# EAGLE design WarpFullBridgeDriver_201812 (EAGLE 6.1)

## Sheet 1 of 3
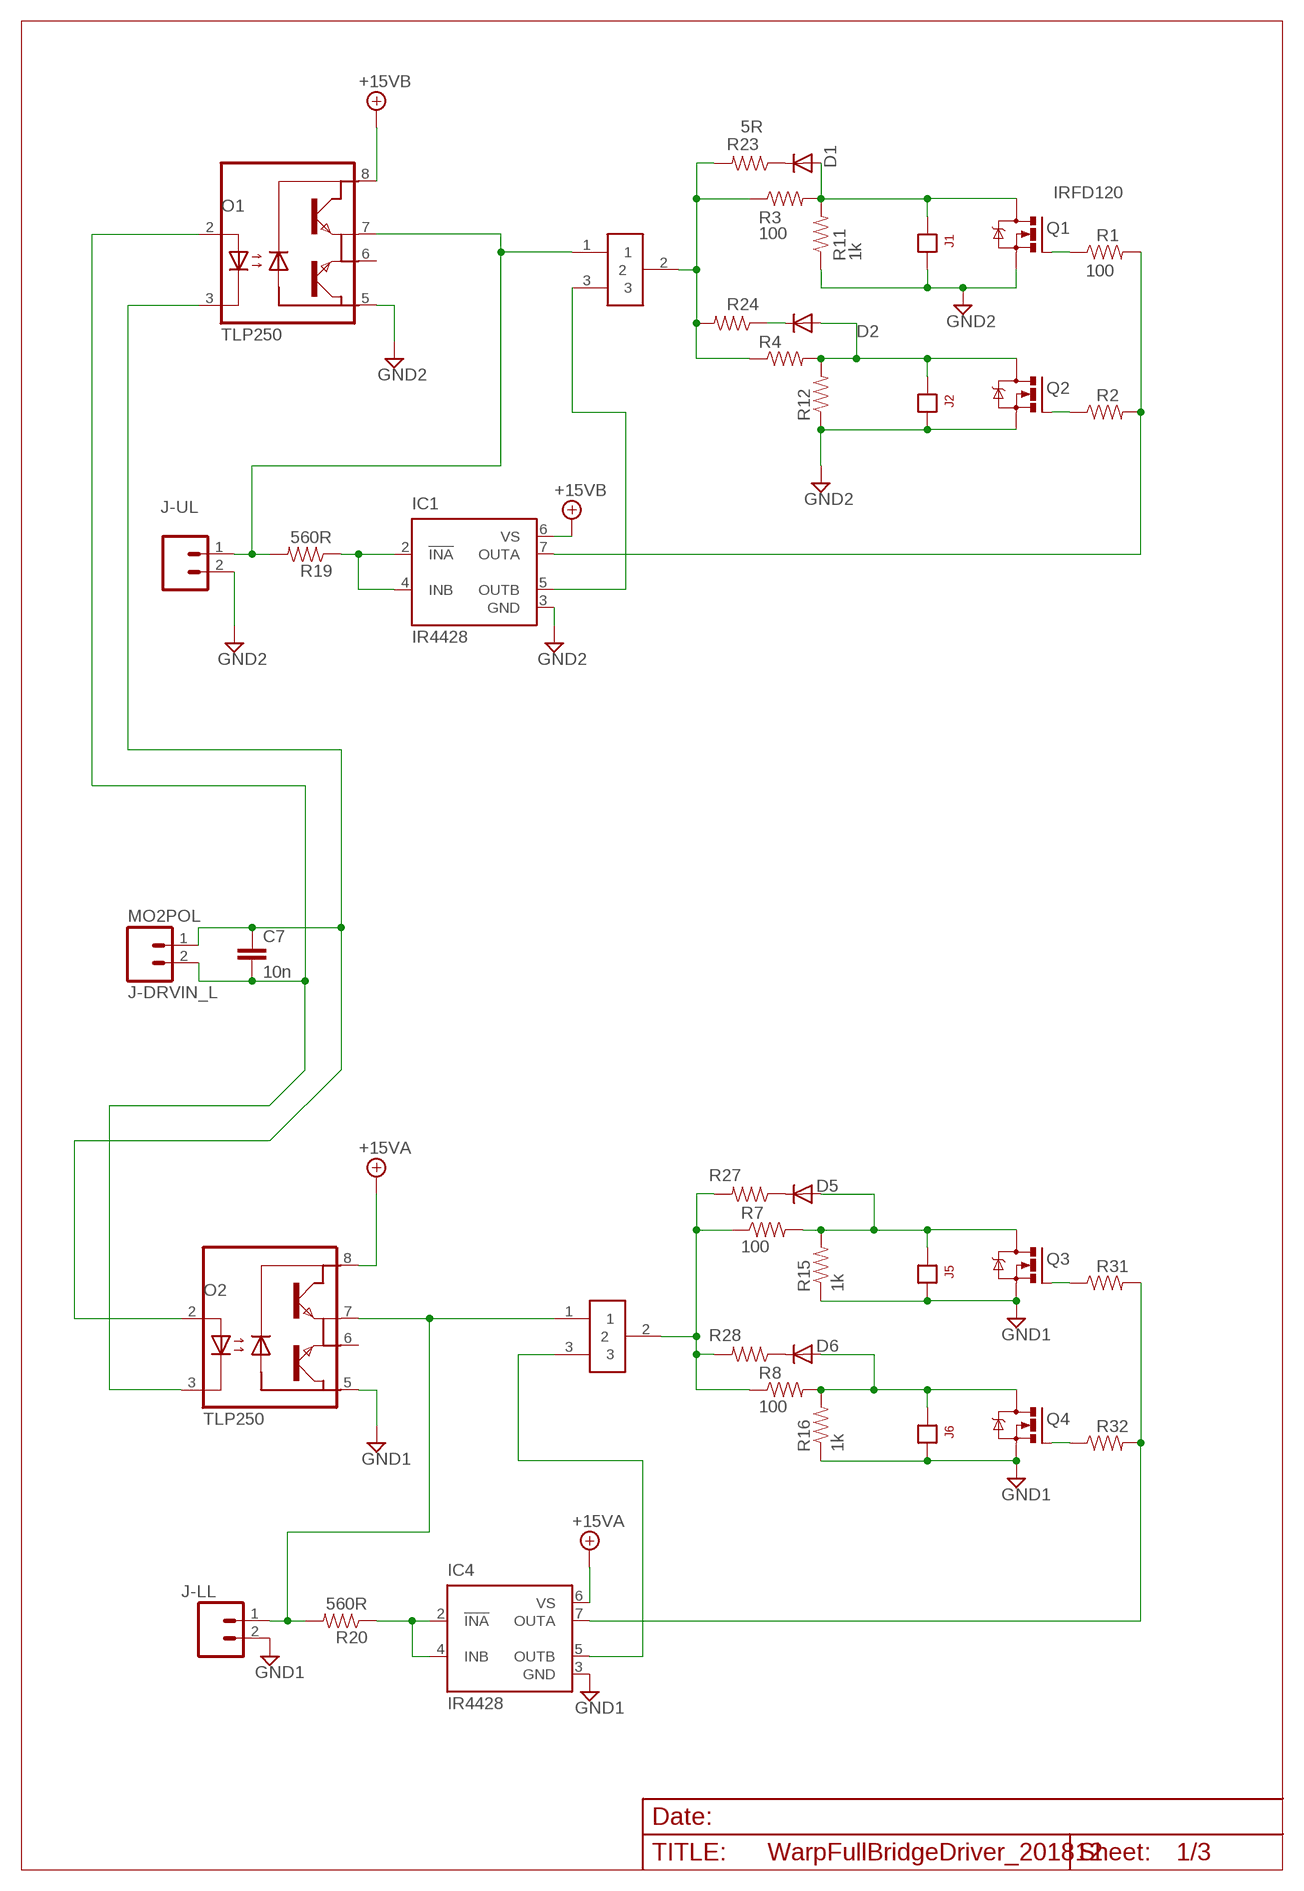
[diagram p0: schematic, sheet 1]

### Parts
C7  10n  BCAP  [BCAP]
D1  1N4148DO35-7  [D3]
D2  1N4148DO35-7  [D3]
D5  1N4148DO35-7  [D3]
D6  1N4148DO35-7  [D3]
IC1  IR4428  [DIL08]
IC4  IR4428  [DIL08]
J1  JP1  [JP1]
J2  JP1  [JP1]
J5  JP1  [JP1]
J6  JP1  [JP1]
J-DRVIN_L  MO2POL  [MOLEX-1X2]
J-LL  MO2POL  [MOLEX-1X2]
J-UL  MO2POL  [MOLEX-1X2]
JP1  JP1X3  [JP1X3]
JP2  JP1X3  [JP1X3]
O1  TLP250  TLP250DIP8-L39  [DIL08-L39]
O2  TLP250  TLP250DIP8-L39  [DIL08-L39]
Q1  IRFD120  [DIL04]
Q2  IRFD120  [DIL04]
Q3  IRFD120  [DIL04]
Q4  IRFD120  [DIL04]
R1  100  RESISTORPTH-1/4W  [AXIAL-0.4]
R2  100  RESISTORPTH-1/4W  [AXIAL-0.4]
R3  100  RESISTORPTH-1/4W  [AXIAL-0.4]
R4  100  RESISTORPTH-1/4W  [AXIAL-0.4]
R7  100  RESISTORPTH-1/4W  [AXIAL-0.4]
R8  100  RESISTORPTH-1/4W  [AXIAL-0.4]
R11  1k  R4  [AXIAL-0.4]
R12  1k  R4  [AXIAL-0.4]
R15  1k  R4  [AXIAL-0.4]
R16  1k  R4  [AXIAL-0.4]
R19  560R  R4  [AXIAL-0.4]
R20  560R  R4  [AXIAL-0.4]
R23  5R  R4  [AXIAL-0.4]
R24  5R  R4  [AXIAL-0.4]
R27  5R  R4  [AXIAL-0.4]
R28  5R  R4  [AXIAL-0.4]
R31  100  RESISTORPTH-1/4W  [AXIAL-0.4]
R32  100  RESISTORPTH-1/4W  [AXIAL-0.4]

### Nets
+15VA: IC4.6(VS) O2.8(VCC) ; also sheet 3
+15VB: IC1.6(VS) O1.8(VCC) ; also sheet 3
GND1: IC4.3(GND) J5.2 J6.2 J-LL.2 O2.5(GND) Q3.4(S) Q4.4(S) R15.P$1 R16.P$1 ; also sheet 3
GND2: IC1.3(GND) J1.2 J2.2 J-UL.2 O1.5(GND) Q1.4(S) Q2.4(S) R11.P$1 R12.P$1 ; also sheet 3
N$1: J-LL.1 JP2.1 O2.7(VO2) R20.P$2
N$2: D2.A J2.1 Q2.1(D) R4.P$2 R12.P$2
N$3: D1.A J1.1 Q1.1(D) R3.P$2 R11.P$2
N$4: D1.C R23.P$1
N$5: J-UL.1 JP1.1 O1.7(VO2) R19.P$2
N$6: IC1.2(!INA) IC1.4(INB) R19.P$1
N$7: Q1.3(G) R1.P$1
N$8: D6.A J6.1 Q4.1(D) R8.P$2 R16.P$2
N$11: C7.1 J-DRVIN_L.1 O1.3(C) O2.2(A)
N$12: D5.A J5.1 Q3.1(D) R7.P$2 R15.P$2
N$15: IC1.7(OUTA) R1.P$2 R2.P$2
N$16: C7.2 J-DRVIN_L.2 O1.2(A) O2.3(C)
N$17: Q2.3(G) R2.P$1
N$21: D2.C R24.P$1
N$23: JP2.2 R7.P$1 R8.P$1 R27.P$2 R28.P$2
N$27: IC1.5(OUTB) JP1.3
N$28: D5.C R27.P$1
N$29: IC4.7(OUTA) R31.P$2 R32.P$2
N$30: IC4.2(!INA) IC4.4(INB) R20.P$1
N$31: D6.C R28.P$1
N$32: IC4.5(OUTB) JP2.3
N$36: JP1.2 R3.P$1 R4.P$1 R23.P$2 R24.P$2
N$39: Q3.3(G) R31.P$1
N$41: Q4.3(G) R32.P$1
Unconnected: O1.6(VO) O2.6(VO)

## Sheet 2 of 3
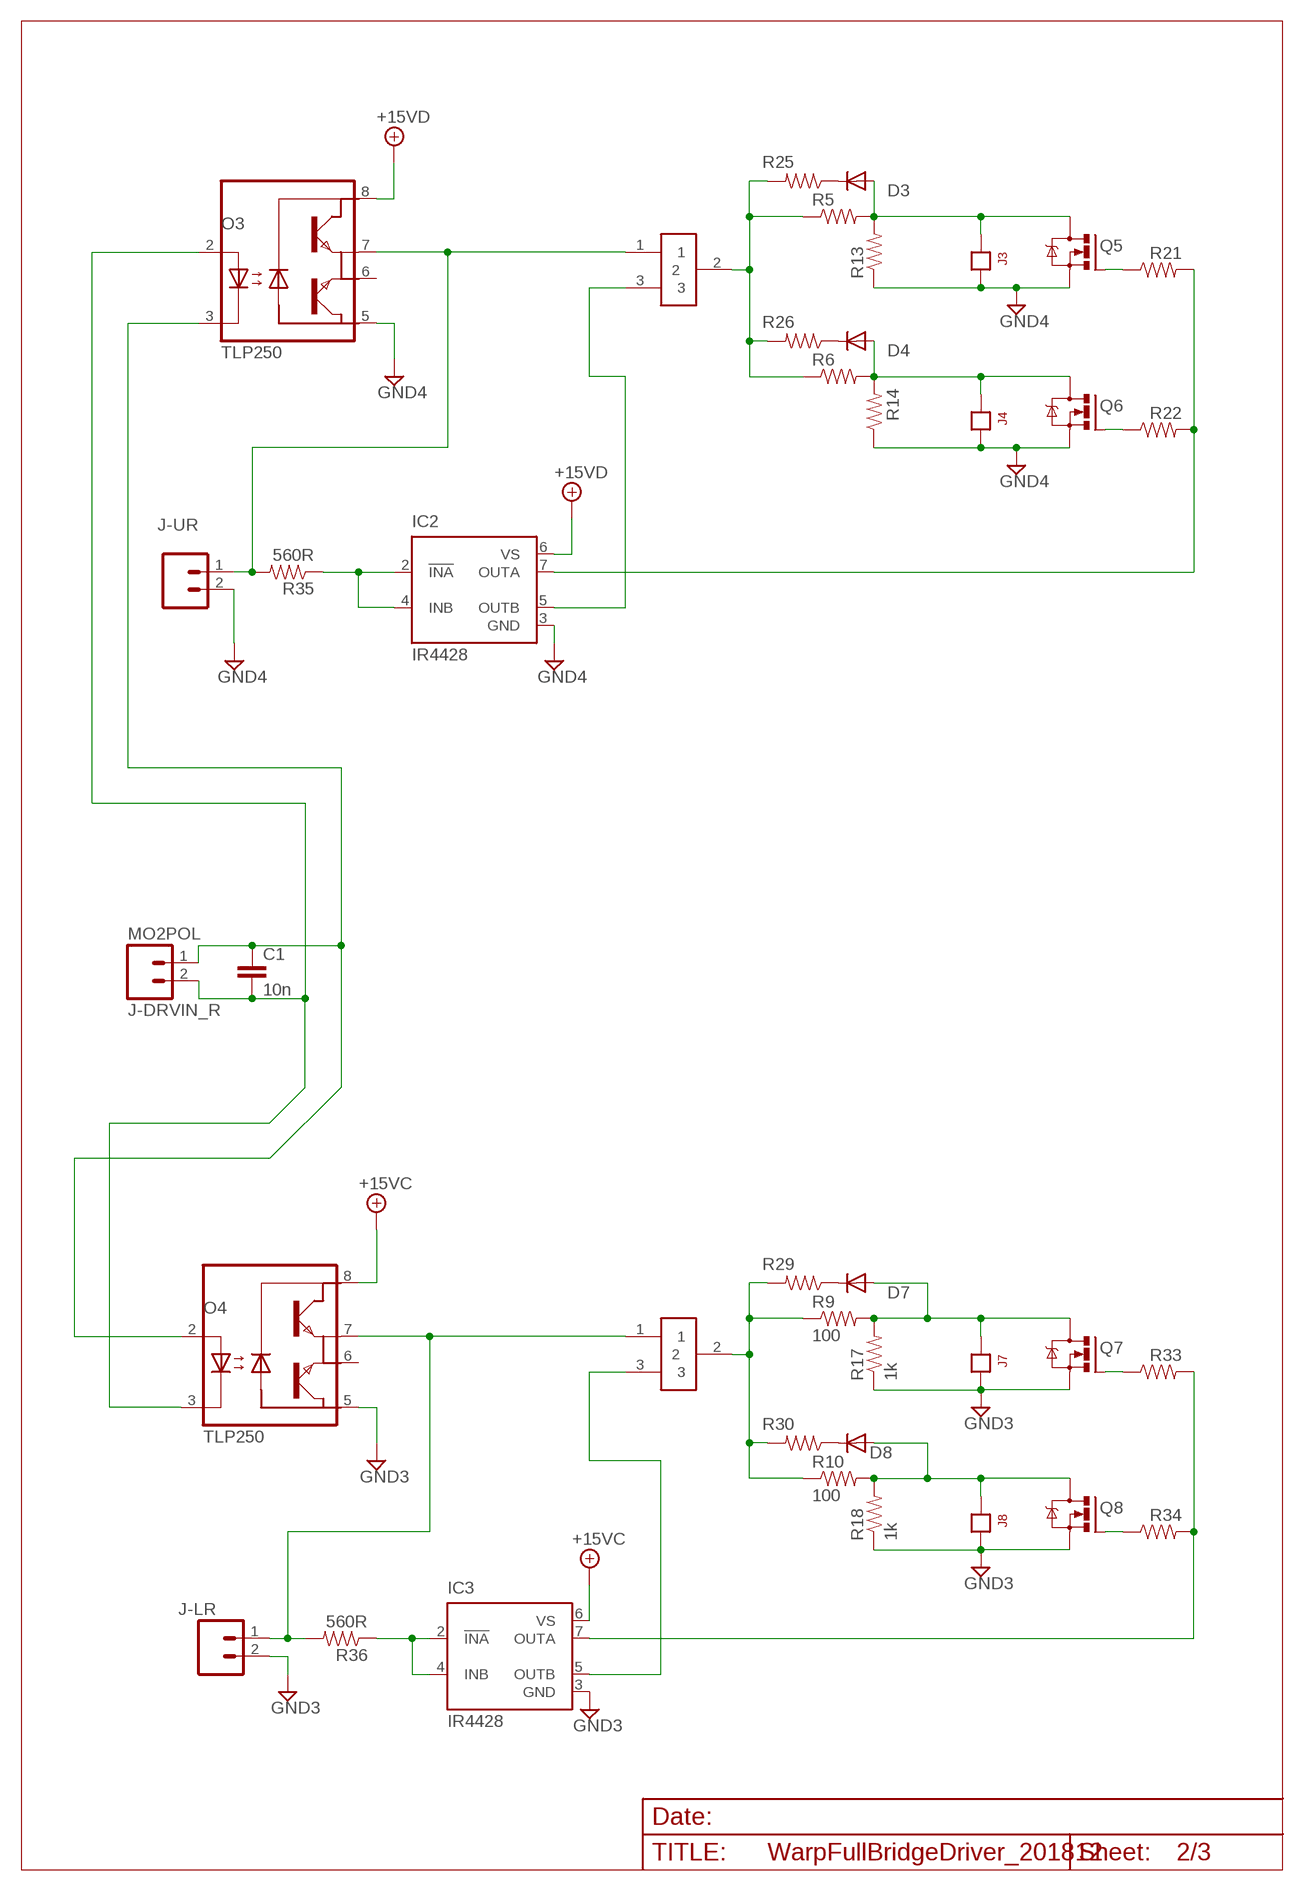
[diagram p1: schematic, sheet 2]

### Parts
C1  10n  BCAP  [BCAP]
D3  1N4148DO35-7  [D3]
D4  1N4148DO35-7  [D3]
D7  1N4148DO35-7  [D3]
D8  1N4148DO35-7  [D3]
IC2  IR4428  [DIL08]
IC3  IR4428  [DIL08]
J3  JP1  [JP1]
J4  JP1  [JP1]
J7  JP1  [JP1]
J8  JP1  [JP1]
J-DRVIN_R  MO2POL  [MOLEX-1X2]
J-LR  MO2POL  [MOLEX-1X2]
J-UR  MO2POL  [MOLEX-1X2]
JP3  JP1X3  [JP1X3]
JP4  JP1X3  [JP1X3]
O3  TLP250  TLP250DIP8-L39  [DIL08-L39]
O4  TLP250  TLP250DIP8-L39  [DIL08-L39]
Q5  IRFD120  [DIL04]
Q6  IRFD120  [DIL04]
Q7  IRFD120  [DIL04]
Q8  IRFD120  [DIL04]
R5  100  RESISTORPTH-1/4W  [AXIAL-0.4]
R6  100  RESISTORPTH-1/4W  [AXIAL-0.4]
R9  100  RESISTORPTH-1/4W  [AXIAL-0.4]
R10  100  RESISTORPTH-1/4W  [AXIAL-0.4]
R13  1k  R4  [AXIAL-0.4]
R14  1k  R4  [AXIAL-0.4]
R17  1k  R4  [AXIAL-0.4]
R18  1k  R4  [AXIAL-0.4]
R21  100  RESISTORPTH-1/4W  [AXIAL-0.4]
R22  100  RESISTORPTH-1/4W  [AXIAL-0.4]
R25  5R  R4  [AXIAL-0.4]
R26  5R  R4  [AXIAL-0.4]
R29  5R  R4  [AXIAL-0.4]
R30  5R  R4  [AXIAL-0.4]
R33  100  RESISTORPTH-1/4W  [AXIAL-0.4]
R34  100  RESISTORPTH-1/4W  [AXIAL-0.4]
R35  560R  R4  [AXIAL-0.4]
R36  560R  R4  [AXIAL-0.4]

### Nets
+15VC: IC3.6(VS) O4.8(VCC) ; also sheet 3
+15VD: IC2.6(VS) O3.8(VCC) ; also sheet 3
GND3: IC3.3(GND) J7.2 J8.2 J-LR.2 O4.5(GND) Q7.4(S) Q8.4(S) R17.P$1 R18.P$1 ; also sheet 3
GND4: IC2.3(GND) J3.2 J4.2 J-UR.2 O3.5(GND) Q5.4(S) Q6.4(S) R13.P$1 R14.P$1 ; also sheet 3
N$9: D3.A J3.1 Q5.1(D) R5.P$2 R13.P$2
N$10: D4.A J4.1 Q6.1(D) R6.P$2 R14.P$2
N$13: D7.A J7.1 Q7.1(D) R9.P$2 R17.P$2
N$14: D8.A J8.1 Q8.1(D) R10.P$2 R18.P$2
N$18: IC2.7(OUTA) R21.P$2 R22.P$2
N$19: Q5.3(G) R21.P$1
N$22: Q6.3(G) R22.P$1
N$24: D3.C R25.P$1
N$25: D4.C R26.P$1
N$26: J-UR.1 JP3.1 O3.7(VO2) R35.P$2
N$33: IC2.5(OUTB) JP3.3
N$34: D7.C R29.P$1
N$35: J-LR.1 JP4.1 O4.7(VO2) R36.P$2
N$37: D8.C R30.P$1
N$38: IC3.5(OUTB) JP4.3
N$40: JP3.2 R5.P$1 R6.P$1 R25.P$2 R26.P$2
N$43: Q7.3(G) R33.P$1
N$44: IC2.2(!INA) IC2.4(INB) R35.P$1
N$45: Q8.3(G) R34.P$1
N$46: IC3.7(OUTA) R33.P$2 R34.P$2
N$47: C1.1 J-DRVIN_R.1 O3.3(C) O4.2(A)
N$48: C1.2 J-DRVIN_R.2 O3.2(A) O4.3(C)
N$49: JP4.2 R9.P$1 R10.P$1 R29.P$2 R30.P$2
N$51: IC3.2(!INA) IC3.4(INB) R36.P$1
Unconnected: O3.6(VO) O4.6(VO)

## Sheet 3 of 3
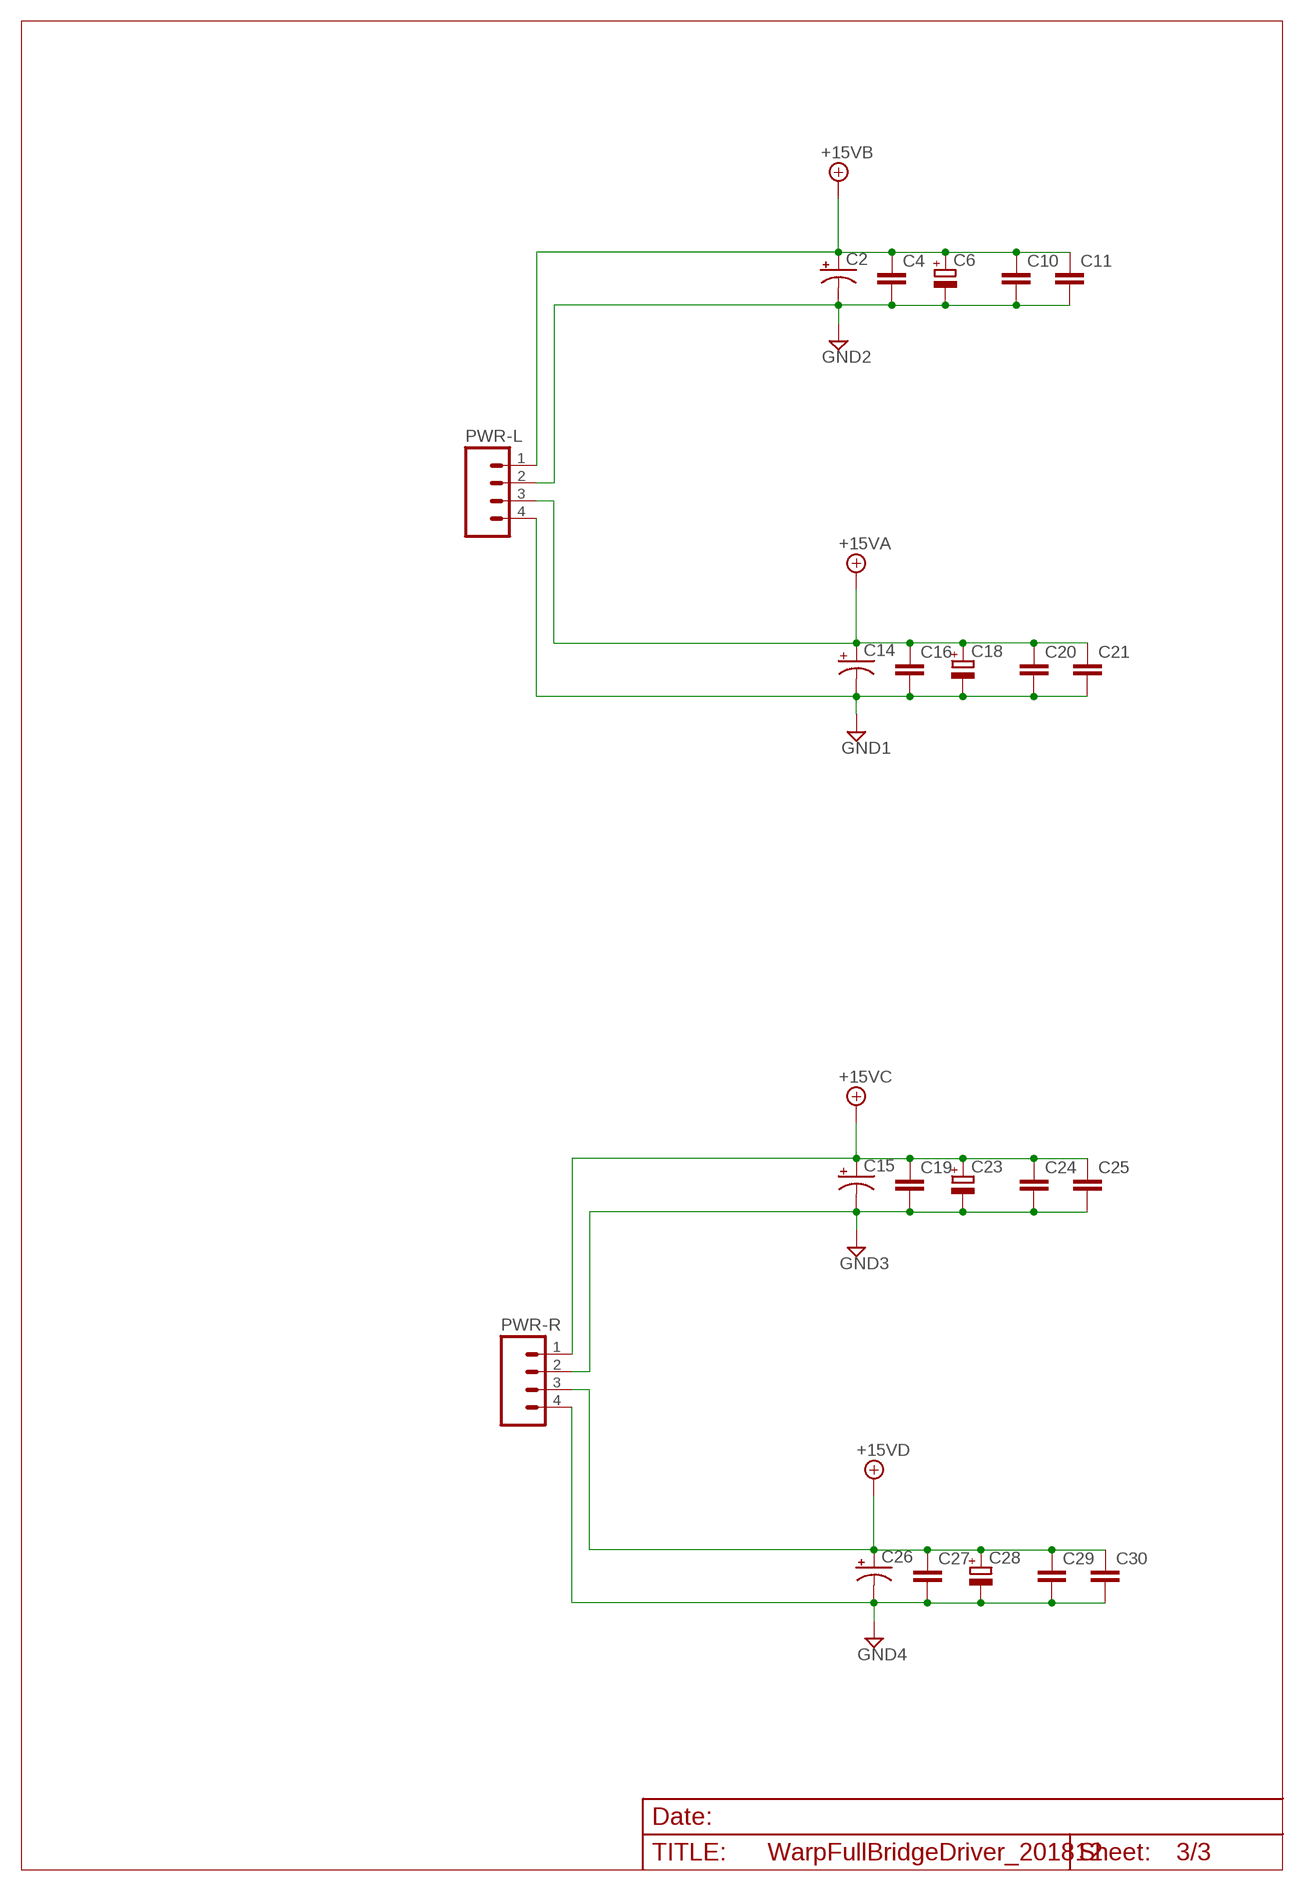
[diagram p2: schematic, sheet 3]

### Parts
C2  CAP_POLPTH1  [CPOL-RADIAL-100UF-25V]
C4  BCAP  [BCAP]
C6  C-RB200100  [CPOL-RADIAL-10UF-25V]
C10  BCAP  [BCAP]
C11  BCAP  [BCAP]
C14  CAP_POLPTH1  [CPOL-RADIAL-100UF-25V]
C15  CAP_POLPTH1  [CPOL-RADIAL-100UF-25V]
C16  BCAP  [BCAP]
C18  C-RB200100  [CPOL-RADIAL-10UF-25V]
C19  BCAP  [BCAP]
C20  BCAP  [BCAP]
C21  BCAP  [BCAP]
C23  C-RB200100  [CPOL-RADIAL-10UF-25V]
C24  BCAP  [BCAP]
C25  BCAP  [BCAP]
C26  CAP_POLPTH1  [CPOL-RADIAL-100UF-25V]
C27  BCAP  [BCAP]
C28  C-RB200100  [CPOL-RADIAL-10UF-25V]
C29  BCAP  [BCAP]
C30  BCAP  [BCAP]
PWR-L  MO4POL  [MOLEX-4]
PWR-R  MO4POL  [MOLEX-4]

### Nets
+15VA: C14.1(+) C16.1 C18.1(+) C20.1 C21.1 PWR-L.3 ; also sheet 1
+15VB: C2.1(+) C4.1 C6.1(+) C10.1 C11.1 PWR-L.1 ; also sheet 1
+15VC: C15.1(+) C19.1 C23.1(+) C24.1 C25.1 PWR-R.1 ; also sheet 2
+15VD: C26.1(+) C27.1 C28.1(+) C29.1 C30.1 PWR-R.3 ; also sheet 2
GND1: C14.2(-) C16.2 C18.2(-) C20.2 C21.2 PWR-L.4 ; also sheet 1
GND2: C2.2(-) C4.2 C6.2(-) C10.2 C11.2 PWR-L.2 ; also sheet 1
GND3: C15.2(-) C19.2 C23.2(-) C24.2 C25.2 PWR-R.2 ; also sheet 2
GND4: C26.2(-) C27.2 C28.2(-) C29.2 C30.2 PWR-R.4 ; also sheet 2

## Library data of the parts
C1 C7 = Andrew junk:BCAP
C2 C14 C15 C26 = SparkFun-Passives:CAP_POL: Capacitor Polarized
C4 C10 C11 C16 C19-C21 C24 C25 C27 C29 C30 = Andrew Misc:BCAP
C6 C18 C23 C28 = Andrew:C-RB200100
D1-D8 = Andrew Misc:1N4148: DIODE
IC1-IC4 = ir:IR4428: DUAL LOW SIDE DRIVER Source: ID4426.pdf; MF: INTERNATIONAL RECTIFIER(IR); MPN: IR4428PBF; OC_FARNELL: 1023268; OC_NEWARK: 19K8464
J1-J8 = Andrew Connectors:JP1
J-DRVIN_L J-DRVIN_R J-LL J-LR J-UL J-UR = Andrew_Connectors:MO2POL
JP1-JP4 = Andrew_Connectors:JP1X3
O1-O4 = Andrew IC:TLP250: HEWLETT PACKARD OPTO COUPLER
PWR-L PWR-R = Andrew_Connectors:MO4POL
Q1-Q8 = Andrew Transistor:IRFD120
R1-R10 R21 R22 R31-R34 = SparkFun-Passives:RESISTOR: Resistor
R11-R20 R23-R30 R35 R36 = Andrew Misc:R4

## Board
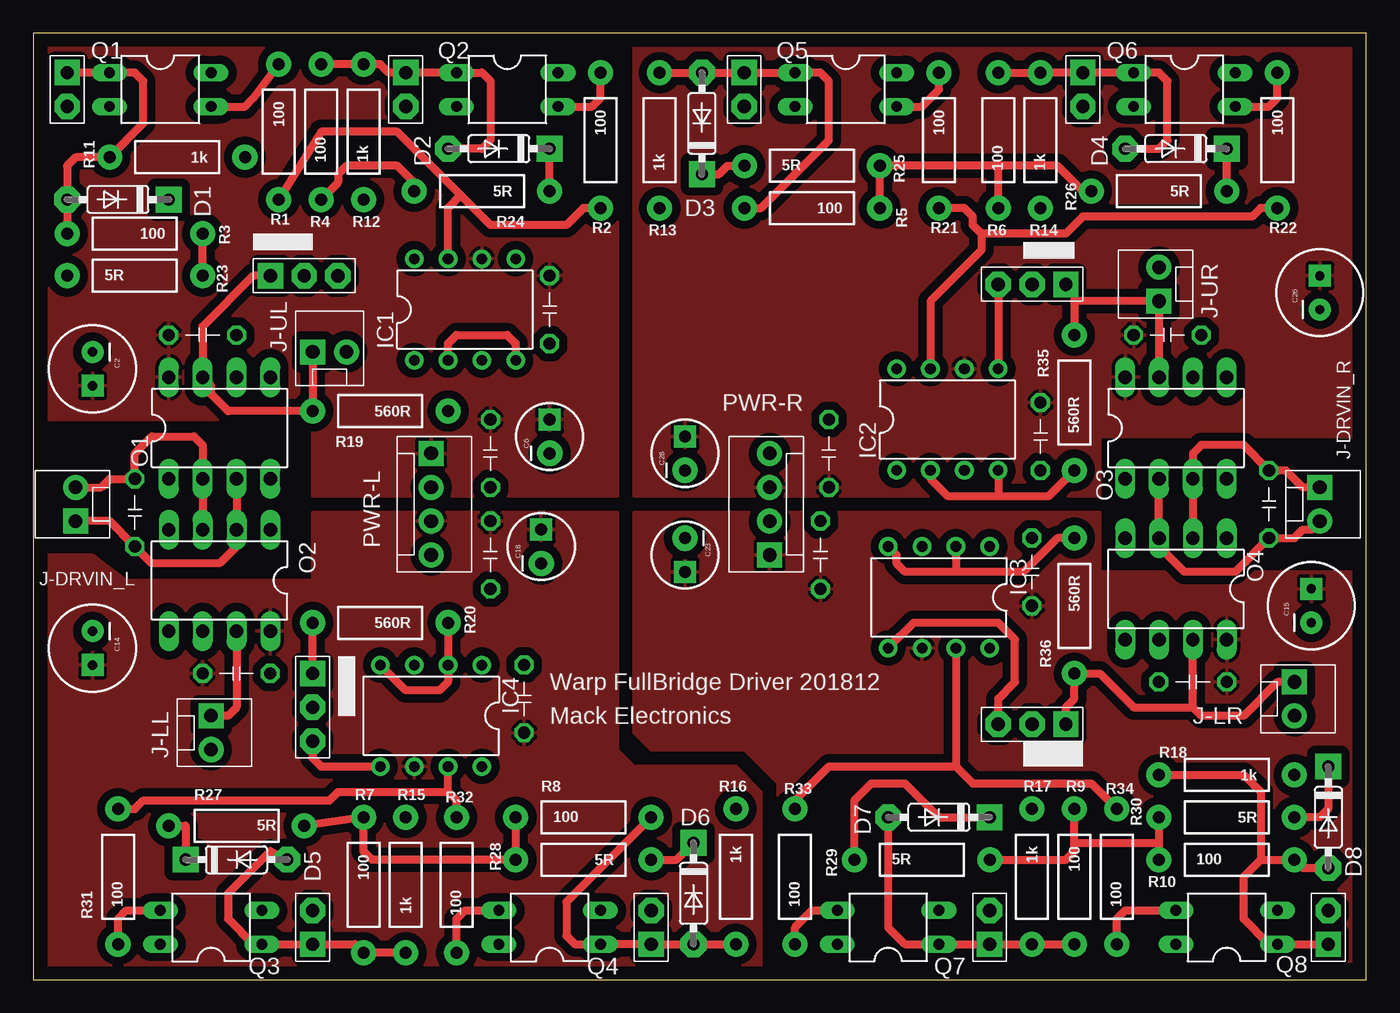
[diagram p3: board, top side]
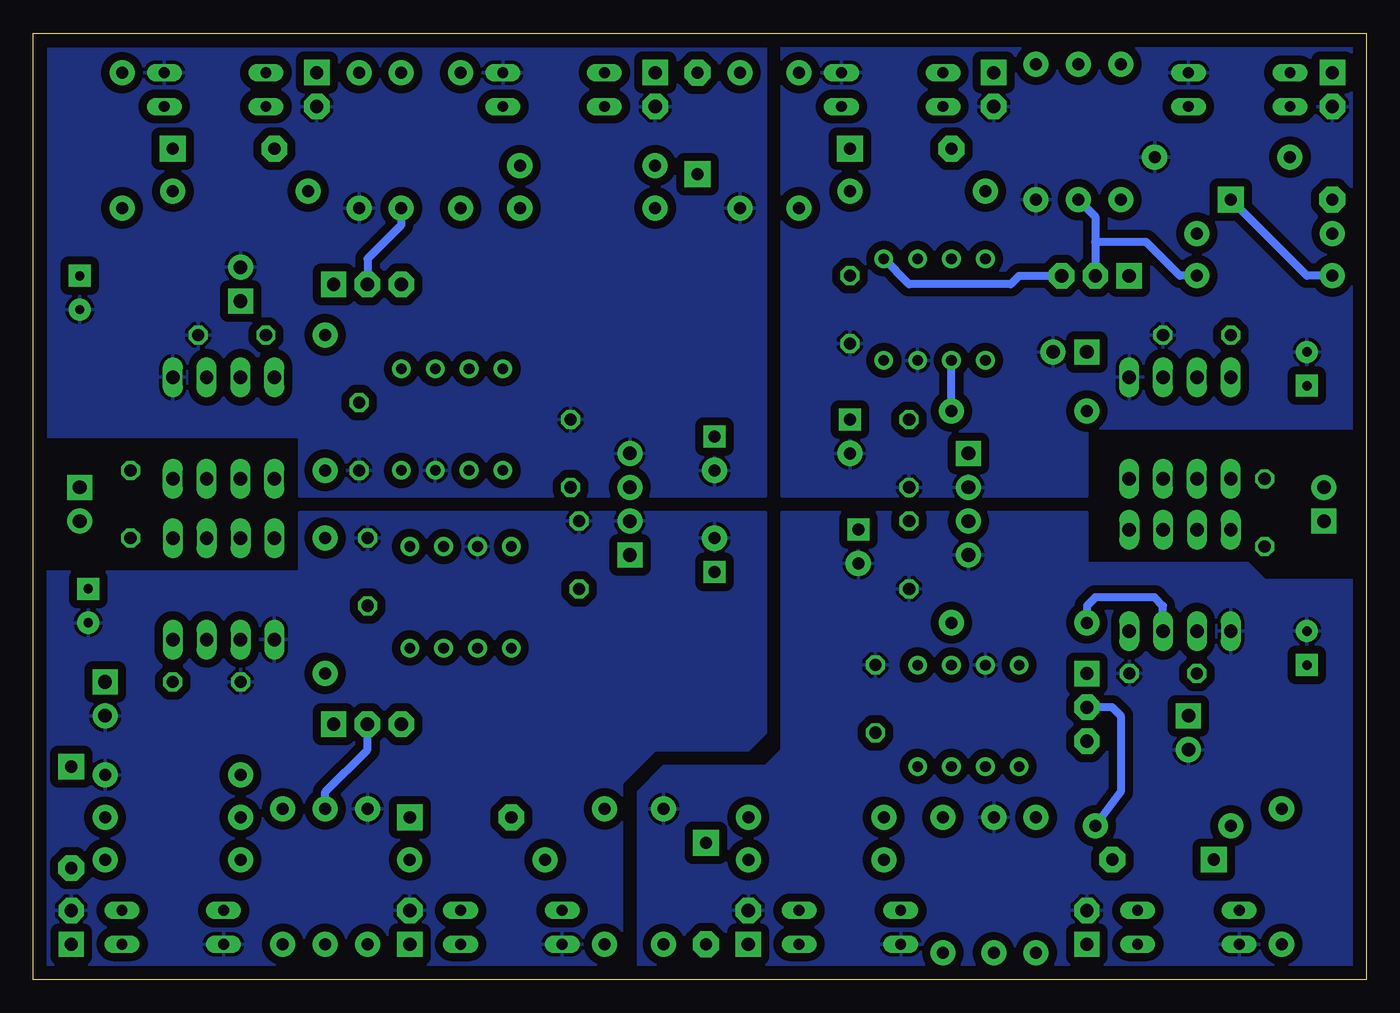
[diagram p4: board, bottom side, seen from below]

Size 100 x 71 mm. Coordinates in mm from the lower left corner, seen from the top.
Outline: 0,0 100,0 100,71 0,71 0,0
Copper layers (1*16): Top 0.035mm / dielectric 1.5mm / Bottom 0.035mm
Design rules: minimum track width 10mil, minimum drill 24mil, track to track 8mil, track to pad 8mil, pad to pad 8mil, via to via 8mil, smd to smd 8mil, copper to edge 40mil, drill to drill 8mil, minimum pad ring 10mil, minimum via ring 8mil, stop-mask expansion 4mil, vias tented up to drill 0mil, thermal gap 10mil

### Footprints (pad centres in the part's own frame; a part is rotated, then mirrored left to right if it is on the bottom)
BCAP = drill 0.914 octagon: 1 -2.54,0; 2 2.54,0
CPOL-RADIAL-100UF-25V = drill 0.7 pad 1.651 square: 1 1.27,0 | drill 0.7 pad 1.651: 2 -1.27,0
CPOL-RADIAL-10UF-25V = drill 0.914 pad 1.651 square: 1 1.27,0 | drill 0.914 pad 1.905: 2 -1.27,0
D3 = drill 0.914 pad 1.93 octagon: A 3.81,0 | drill 0.914 pad 1.93 square: C -3.81,0
DIL08 = drill 0.8 pad 1.4: 1 -3.81,-3.81; 2 -1.27,-3.81; 3 1.27,-3.81; 4 3.81,-3.81; 5 3.81,3.81; 6 1.27,3.81; 7 -1.27,3.81; 8 -3.81,3.81
JP1 = drill 1 pad 1.905 square: 1 -1.27,0 | drill 1 pad 1.905 octagon: 2 1.27,0
MOLEX-1X2 = drill 1.016 pad 1.88 square: 1 0,0 | drill 1.016 pad 1.88: 2 2.54,0
JP1X3 = drill 1 pad 1.905 square: 1 -2.54,0 | drill 1 pad 1.905 octagon: 2 0,0; 3 2.54,0
DIL08-L39 = drill 1 long: 1 -3.81,-3.81; 2 -1.27,-3.81; 3 1.27,-3.81; 4 3.81,-3.81; 5 3.81,3.81; 6 1.27,3.81; 7 -1.27,3.81; 8 -3.81,3.81
MOLEX-4 = drill 1.016 pad 1.88 square: 1 -3.81,0 | drill 1.016 pad 1.88: 2 -1.27,0; 3 1.27,0; 4 3.81,0
DIL04 = drill 0.813 long: 1 -1.27,-3.81; 2 1.27,-3.81; 3 1.27,3.81; 4 -1.27,3.81
AXIAL-0.4 = drill 0.9 pad 1.88: P$1 -5.08,0; P$2 5.08,0

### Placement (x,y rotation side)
C1  92.71,35.66 270 top
C2  4.45,45.83 270 top
C4  12.7,48.37 0 top
C6  38.73,40.74 90 top
C7  7.62,35.03 90 top
C10  38.73,50.27 270 top
C11  34.29,39.48 270 top
C14  4.45,24.87 270 top
C15  95.89,28.05 90 top
C16  36.83,21.06 90 top
C18  38.1,32.49 90 top
C19  87,22.33 180 top
C20  34.29,31.85 270 top
C21  15.24,22.97 0 top
C23  48.9,31.85 270 top
C24  74.93,30.59 90 top
C25  59.05,31.85 90 top
C26  96.52,51.54 90 top
C27  85.09,48.37 0 top
C28  48.9,39.48 90 top
C29  59.69,39.48 90 top
C30  75.56,40.74 270 top
D1  6.35,58.53 180 top
D2  34.92,62.33 180 top
D3  50.16,64.24 90 top
D4  85.72,62.33 180 top
D5  15.24,9 0 top
D6  49.53,6.45 270 top
D7  67.94,12.17 180 top
D8  97.16,12.17 270 top
IC1  32.38,50.27 0 top
IC2  68.58,42.02 0 top
IC3  67.94,28.68 180 top
IC4  29.84,19.79 180 top
J1  2.54,66.78 270 top
J2  27.94,66.78 270 top
J3  53.34,66.78 270 top
J4  78.74,66.78 270 top
J5  20.95,3.91 90 top
J6  46.35,3.91 90 top
J7  71.75,3.91 90 top
J8  97.16,3.91 90 top
J-DRVIN_L  3.17,34.4 90 top
J-DRVIN_R  96.52,36.94 270 top
J-LL  13.34,19.79 270 top
J-LR  94.61,22.33 270 top
J-UL  20.95,47.09 0 top
J-UR  84.45,50.91 90 top
JP1  20.32,52.81 0 top
JP2  20.95,20.42 270 top
JP3  74.93,52.17 180 top
JP4  74.93,19.16 180 top
O1  13.97,41.38 0 top
O2  13.97,29.95 180 top
O3  85.72,41.38 0 top
O4  85.72,29.31 180 top
PWR-L  29.84,35.66 270 top
PWR-R  55.24,35.66 90 top
Q1  9.53,66.78 270 top
Q2  35.56,66.78 270 top
Q3  13.34,3.91 90 top
Q4  38.73,3.91 90 top
Q5  60.96,66.78 270 top
Q6  86.36,66.78 270 top
Q7  64.14,3.91 90 top
Q8  89.53,3.91 90 top
R1  18.41,63.61 270 top
R2  42.55,62.97 270 top
R3  7.62,55.98 180 top
R4  21.59,63.61 90 top
R5  58.42,57.89 180 top
R6  72.39,62.97 90 top
R7  24.77,7.09 270 top
R8  41.27,12.17 0 top
R9  78.11,7.73 270 top
R10  89.53,9 0 top
R11  10.79,61.7 180 top
R12  24.77,63.61 90 top
R13  46.99,62.97 90 top
R14  75.56,62.97 90 top
R15  27.94,7.09 270 top
R16  52.7,7.73 270 top
R17  74.93,7.73 270 top
R18  89.53,15.34 180 top
R19  26.04,42.65 180 top
R20  26.04,26.77 180 top
R21  67.94,62.97 270 top
R22  93.34,62.97 270 top
R23  7.62,52.81 0 top
R24  33.66,59.16 180 top
R25  58.42,61.06 0 top
R26  84.45,59.16 180 top
R27  15.24,11.54 0 top
R28  41.27,9 180 top
R29  66.67,9 0 top
R30  89.53,12.17 180 top
R31  6.35,7.73 90 top
R32  31.75,7.09 90 top
R33  57.15,7.73 90 top
R34  81.28,7.73 90 top
R35  78.11,43.28 90 top
R36  78.11,28.05 270 top

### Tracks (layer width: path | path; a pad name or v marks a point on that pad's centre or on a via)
+15VA
  pour Top (isolate 0.61): 0.64,0.74 0.64,31.85 4.45,31.85 6.99,29.95 20.95,29.95 20.95,35.03 43.81,35.03 43.81,17.25 45.09,15.98 52.7,15.98 54.61,14.07 54.61,0.74
+15VB
  pour Top (isolate 0.61): 0.64,70.59 43.81,70.59 43.81,36.3 20.95,36.3 20.95,42.02 0.64,42.02
+15VC
  pour Top (isolate 0.61): 45.09,35.03 80.01,35.03 80.01,30.59 99.06,30.59 99.06,1.38 55.88,1.38 55.88,14.71 53.34,17.25 46.35,17.25 45.09,18.52
+15VD
  pour Top (isolate 0.61): 45.09,36.3 45.09,69.95 99.06,69.95 99.06,40.74 80.01,40.74 80.01,36.3
GND1
  pour Bottom (isolate 0.61): 0.64,0.74 0.64,29.95 7.62,29.95 8.89,31.22 20.95,31.22 20.95,35.03 43.81,35.03 43.81,17.25 45.09,15.98 52.7,15.98 54.61,14.07 54.61,0.74
GND2
  pour Bottom (isolate 0.61): 0.64,70.59 43.81,70.59 43.81,36.3 20.95,36.3 20.95,37.57 20.95,41.38 0.64,41.38
GND3
  pour Bottom (isolate 0.61): 45.09,35.03 80.01,35.03 80.01,30.59 99.69,30.59 99.69,0.74 55.88,0.74 55.88,14.71 53.34,17.25 46.35,17.25 45.09,18.52
GND4
  pour Bottom (isolate 0.61): 45.09,36.3 45.09,69.95 99.06,69.95 99.06,40.74 80.01,40.74 80.01,36.3
N$1
  Top 0.61: JP2.1 R20.P$2 | O2.7 15.24,20.42 14.61,19.79 J-LL.1
  Bottom 0.61: O2.7 15.24,28.05 15.88,28.68 20.32,28.68 20.95,28.05 R20.P$2
N$2
  Top 0.61: R4.P$2 R12.P$2 26.04,68.69 26.67,68.05 J2.1 Q2.1 33.66,68.05 34.29,67.42 34.29,62.97 33.66,62.33 D2.A
N$3
  Top 0.61: J1.1 Q1.1 7.62,68.05 8.26,67.42 8.26,64.24 R11.P$2 3.17,61.7 2.54,61.06 D1.A R3.P$2
N$4
  Bottom 0.61: R23.P$1 4.45,52.81 D1.C
N$5
  Top 0.61: JP1.1 16.51,52.81 12.7,49 O1.7 13.34,44.55 13.34,43.92 14.61,42.65 R19.P$2 J-UL.1
N$6
  Top 0.61: IC1.2 31.11,47.73 31.75,48.37 35.56,48.37 36.2,47.73 IC1.4
  Bottom 0.61: R19.P$1 IC1.2
N$7
  Top 0.61: Q1.3 15.88,65.51 16.51,66.14 R1.P$1
N$8
  Top 0.61: R16.P$2 D6.A J6.1 Q4.1 40.64,2.64 40.01,3.28 40.01,5.82 R8.P$2
N$9
  Top 0.61: R13.P$2 D3.A J3.1 Q5.1 59.05,68.05 59.69,67.42 59.69,62.97 54.61,57.89 R5.P$2
N$10
  Top 0.61: R6.P$2 R14.P$2 J4.1 Q6.1 84.45,68.05 85.09,67.42 85.09,62.97 84.45,62.33 D4.A
N$11
  Top 0.61: O1.3 O2.2 15.24,32.49 13.97,31.22 8.89,31.22 C7.1 5.71,34.4 J-DRVIN_L.1
N$12
  Top 0.61: R15.P$2 R7.P$2 24.13,2.64 J5.1 Q3.1 16.51,2.64 14.61,4.55 14.61,6.45 17.78,9.63 D5.A
N$13
  Top 0.61: R9.P$2 R17.P$2 J7.1 Q7.1 65.41,2.64 64.14,3.91 D7.A
N$14
  Top 0.61: J8.1 96.52,2.64 Q8.1 92.71,2.64 90.81,4.55 90.81,7.73 92.08,9 | 92.08,9 R10.P$2 95.25,8.36 D8.A | R18.P$2 90.81,15.34 92.08,14.07 92.08,9
N$15
  Top 0.61: R2.P$2 41.27,57.89 40.01,56.62 34.29,56.62 32.07,58.84 | 32.07,58.84 27.3,63.61 21.59,63.61 R1.P$2 | IC1.7 31.11,57.89 32.07,58.84
N$16
  Top 0.61: J-DRVIN_L.2 5.08,36.94 5.71,37.57 C7.2 7.62,39.48 8.89,40.74 12.06,40.74 12.7,40.11 O1.2 O2.3
N$17
  Top 0.61: Q2.3 41.91,65.51 42.55,66.14 R2.P$1
N$18
  Top 0.61: R22.P$2 92.08,57.89 91.44,57.25 78.74,57.25 77.47,55.98 71.12,55.98 | 71.12,55.98 70.48,56.62 70.48,57.25 69.85,57.89 R21.P$2 | 71.12,55.98 71.12,54.72 67.31,50.91 IC2.7
N$19
  Top 0.61: Q5.3 66.67,65.51 67.94,66.78 R21.P$1
N$21
  Top 0.61: R24.P$1 D2.C
N$22
  Top 0.61: Q6.3 92.71,65.51 93.34,66.14 R22.P$1
N$23
  Top 0.61: R27.P$2 R7.P$1 24.77,9.63 25.4,9 R28.P$2 R8.P$1
  Bottom 0.61: R27.P$2 18.41,14.07 18.41,19.79 19.05,20.42 JP2.2
N$24
  Top 0.61: D3.C 51.44,60.43 52.07,61.06 R25.P$1
N$25
  Top 0.61: R26.P$1 D4.C
N$26
  Top 0.61: JP3.1 78.11,51.54 78.11,50.91 | 78.11,50.91 R35.P$2 | 78.11,50.91 J-UR.1 O3.7
N$27
  Bottom 0.61: JP1.3 26.04,52.81 26.67,52.17 34.29,52.17 IC1.5
N$28
  Top 0.61: R27.P$1 11.43,11.54 D5.C
N$29
  Top 0.61: R31.P$2 7.62,12.8 8.26,13.44 22.23,13.44 22.86,14.07 31.11,14.07 | 31.11,14.07 IC4.7 | R32.P$2 31.75,13.44 31.11,14.07
N$30
  Top 0.61: R20.P$1 IC4.2 31.11,22.33 30.48,21.7 27.94,21.7 IC4.4
N$31
  Top 0.61: R28.P$1 48.26,9 D6.C
N$32
  Top 0.61: JP2.3 20.95,16.61 21.59,15.98 IC4.5
N$33
  Top 0.61: JP3.3 IC2.5
N$34
  Top 0.61: R29.P$1 61.59,13.44 62.87,14.71 65.41,14.71 67.94,12.17 D7.C
N$35
  Top 0.61: JP4.1 77.47,20.42 78.11,21.06 R36.P$2 80.01,22.97 82.55,20.42 87,20.42 | 87,20.42 O4.7 | J-LR.1 93.34,22.33 90.81,19.79 87.63,19.79 87,20.42
N$36
  Top 0.61: R24.P$2 28.57,59.8 27.3,61.06 23.5,61.06 22.86,60.43 22.86,59.8 R4.P$1 | R23.P$2 R3.P$1
  Bottom 0.61: R4.P$1 20.32,57.25 20.32,55.35 | 20.32,55.35 JP1.2 | R23.P$2 13.97,52.81 16.51,55.35 20.32,55.35
N$37
  Top 0.61: D8.C 97.16,12.8 96.52,12.17 R30.P$1
N$38
  Top 0.61: JP4.3 72.39,21.06 73.66,22.33 73.66,25.51 72.39,26.77 66.04,26.77 IC3.5
N$39
  Top 0.61: R31.P$1 6.35,4.55 6.99,5.18 Q3.3
N$40
  Top 0.61: R5.P$1 R25.P$2 72.39,61.06 | R6.P$1 72.39,61.06 | R26.P$2 78.74,59.16 76.83,61.06 72.39,61.06
  Bottom 0.61: R6.P$1 72.39,56.62 74.93,54.08 JP3.2
N$41
  Top 0.61: R32.P$1 31.75,4.55 32.38,5.18 Q4.3
N$43
  Top 0.61: R33.P$1 57.15,3.91 58.42,5.18 Q7.3
N$44
  Top 0.61: IC2.2 67.31,37.57 68.58,36.3 72.39,36.3 | 72.39,36.3 76.2,36.3 R35.P$1 | IC2.4 72.39,36.3
N$45
  Top 0.61: R34.P$1 81.28,4.55 81.92,5.18 Q8.3
N$46
  Top 0.61: R33.P$2 57.15,13.44 59.69,15.98 69.22,15.98 | 69.22,15.98 70.48,14.71 79.38,14.71 R34.P$2 | IC3.7 69.22,15.98
N$47
  Top 0.61: O4.2 O3.3 87,39.48 87.63,40.11 90.81,40.11 C1.1 93.98,38.2 95.25,36.94 J-DRVIN_R.1
N$48
  Top 0.61: O3.2 O4.3 84.45,32.49 86.36,30.59 90.17,30.59 C1.2 94.61,33.12 95.25,33.76 95.89,33.76 J-DRVIN_R.2
N$49
  Top 0.61: R30.P$2 84.45,10.27 | 84.45,10.27 R10.P$1 | 78.11,10.27 84.45,10.27 | R29.P$2 77.47,9 78.11,9.63 78.11,10.27 | 78.11,10.27 R9.P$1
  Bottom 0.61: R9.P$1 78.11,14.07 74.93,17.25 JP4.2
N$51
  Top 0.61: R36.P$1 76.83,33.12 74.3,30.59 69.22,30.59 | 69.22,30.59 65.41,30.59 64.77,31.22 64.77,31.85 IC3.4 | IC3.2 69.22,30.59

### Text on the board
tPlace: Warp FullBridge Driver 201812 | Mack Electronics

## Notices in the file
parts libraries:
SparkFun-Passives: Licensing: CC v3.0 Share-Alike You are welcome to use this library for commercial purposes.
